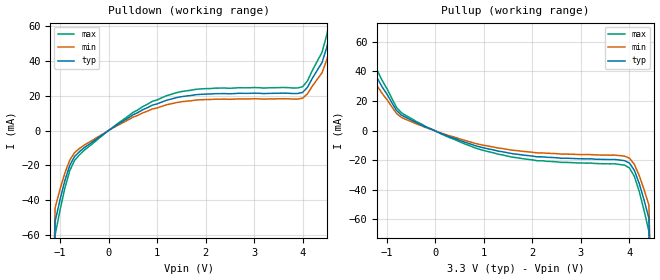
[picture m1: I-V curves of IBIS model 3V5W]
[IBIS Ver]   2.1
[File name]   5811_3.ibs
[File Rev]   2.0
[Date]   1/5/2005
[Source]   ICS MicroClock Applications Engineering 2
[Disclaimer] This information is for modeling purposes only, and is
(C) Copyright Integrated Circuit Systems, Inc. 1997-2005
   All rights reserved
ICS hereby grants the user of this IBIS model a non-exclusive,
nontransferable license to use this IBIS model under the following terms.
Before using this IBIS model, the user should read this license.
If the user does not accept these terms,  the IBIS model should be
returned to ICS within 30 days.
   The user is granted this license only to use the IBIS model and
is not granted rights to sell, load, rent, lease or license the IBIS
model in whole or in part, or in modified form to anyone other than
user. User may modify the IBIS model to suit its specific
applications but rights to derivative works and such modifications
shall belong to ICS.
   This IBIS model is provided on an "AS IS" basis and ICS makes
absolutely no warranty with respect to the information contained
herein. ICS DISCLAIMS AND CUSTOMER WAIVES ALL WARRANTIES, EXPRESS
OR IMPLIED, INCLUDING WARRANTIES OF MERCHANTABILITY OR FITNESS FOR
A PARTICULAR PURPOSE. The entire risk as to quality and performance
is with the Customer. ACCORDINGLY, IN NO EVENT SHALL THE COMPANY BE
LIABLE FOR ANY DAMAGES, WHETHER IN CONTRACT OR TORT,INCLUDING ANY
LOST PROFITS OR OTHER INCIDENTAL, CONSEQUENTIAL, EXEMPLARY, OR
PUNITIVE DAMAGES ARISING OUT OF THE USE OR APPLICATION OF THE IBIS
model provided in this package. Further, ICS reserves the right to
make changes without notice to any product herein to improve
reliability, function, or design. ICS does not convey any license
under patent rights or any other intellectual property rights,
including those of third parties.
   ICS is not obligated to provide maintenance or support
for the licensed IBIS model.
[Component]   MK5811
[Manufacturer] Integrated Circuit Systems Inc.
[Package]
|   typ   min   max
R_pkg   40m   35m   45m
L_pkg   1.65nH   1.35nH   1.95nH
C_pkg   0.24pF   0.14pF   0.34pF
[pin]   signal_name   model_name   R_pin   L_pin   C_pin
   5   SSCLK   3V5W
| Models and submodels in the file (1): 3V5W (Output)
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|   MK5811 3.3V Clock Drive Model
| This model is suitable for the output pins on the
| MK5811
[Model]   3V5W
Model_type   Output
Polarity   Non-Inverting
|   typ   min   max
C_comp   5pF   4pF   6pF
|   typ   min   max
[Voltage range]   3.3V   3.0V   3.63V
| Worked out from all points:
|   slope of the pulldown table from 0 to 0.495 V, typ, clamps not added: 56 ohm
|   slope of the pullup table from 0 to 0.495 V, typ, clamps not added: 78.9 ohm
[pulldown]
|Voltage I (typ)   I (min)   I (max)
-3.3V     -3A        -3A        -3A
-1.1V     -51.94mA   -44.15mA   -59.73mA
-900mV    -28.66mA   -24.36mA   -32.95mA
-800mV    -20.05mA   -17.04mA   -23.06mA
-700mV    -14.87mA   -12.64mA   -17.1mA
700mV     11.82mA    10.05mA    13.6mA
1.8V      20.5mA     17.42mA    23.58mA
4V        21.79mA    18.52mA    25.06mA
4.4V      38.86mA    33.03mA    44.68mA
4.5V      47.83mA    40.65mA    55mA
4.6V      59.8mA     50.83mA    68.78mA
6.6V      3A         3A         3A
[pullup]
|Voltage I (typ)   I (min)   I (max)
-3.3V     3A         3A         3A
-1.4V     59.82mA    50.85mA    68.8mA
-1.2V     35.52mA    30.19mA    40.84mA
-800mV    13.55mA    11.52mA    15.58mA
-200mV    2.372mA    2.016mA    2.728mA
800mV     -10.03mA   -8.53mA    -11.54mA
1.6V      -15.73mA   -13.37mA   -18.09mA
3.9V      -20.39mA   -17.33mA   -23.45mA
4.1V      -26.93mA   -22.89mA   -30.97mA
4.2V      -35.77mA   -30.4mA    -41.13mA
4.4V      -59.34mA   -50.44mA   -68.25mA
6.6V      -3A        -3A        -3A
[Ramp]
|   typ   min   max
dV/dt_r   0.53/0.30n   0.50/0.33n   0.56/0.27n
dV/dt_f   0.65/0.33n   0.62/0.36n   0.69/0.30n
